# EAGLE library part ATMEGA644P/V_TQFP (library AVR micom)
ATMEGA644P TQFP pacage AVR micon series. producted by ATMEL.Co
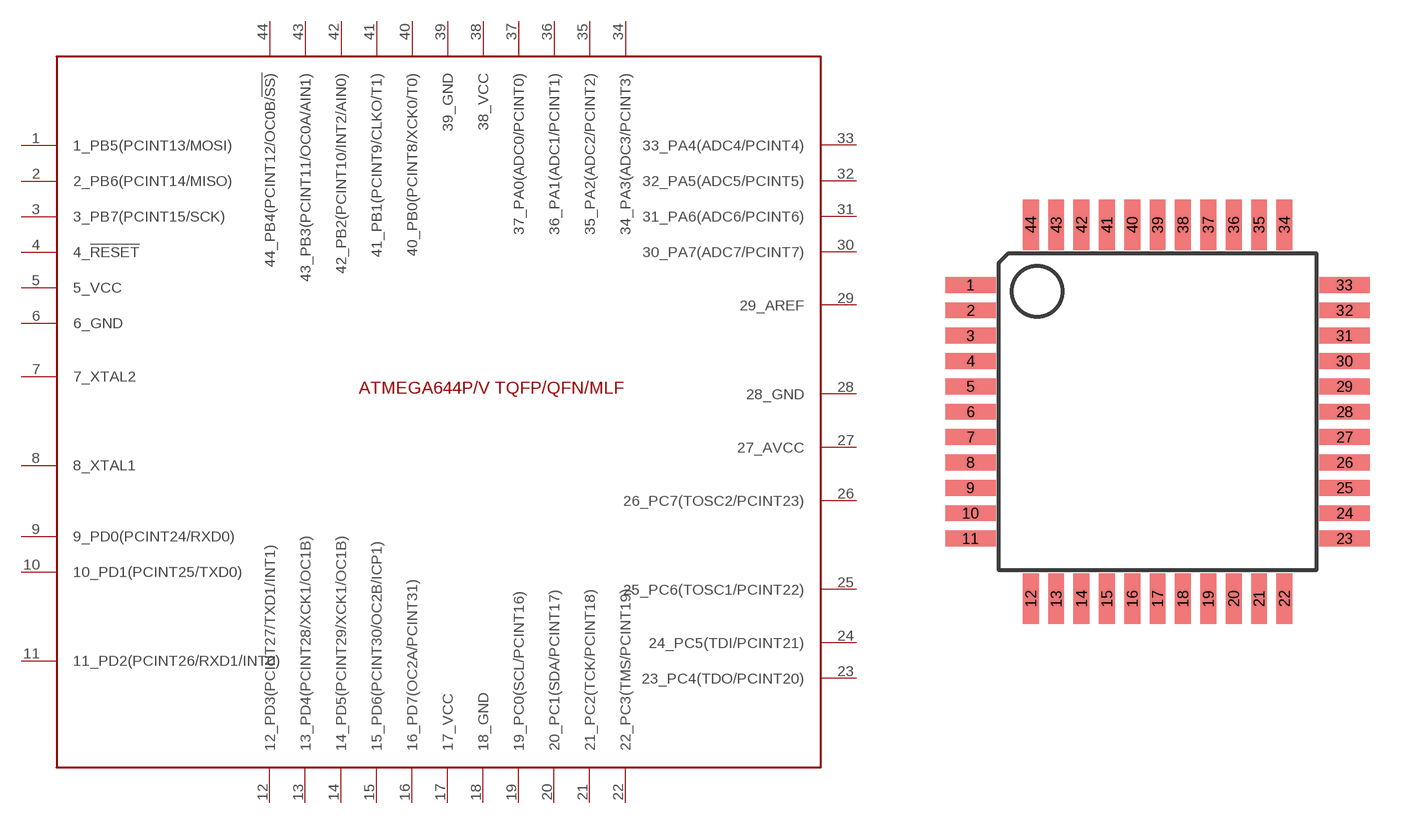
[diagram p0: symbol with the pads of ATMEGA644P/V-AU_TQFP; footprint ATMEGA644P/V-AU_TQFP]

Designator prefix U

## ATMEGA644P/V_TQFP  [ATMEGA644P/V-AU_TQFP]
1  1_PB5(PCINT13/MOSI)
2  2_PB6(PCINT14/MISO)
3  3_PB7(PCINT15/SCK)
4  4_!RESET
5  5_VCC
6  6_GND
7  7_XTAL2
8  8_XTAL1
9  9_PD0(PCINT24/RXD0)
10  10_PD1(PCINT25/TXD0)
11  11_PD2(PCINT26/RXD1/INT0)
12  12_PD3(PCINT27/TXD1/INT1)
13  13_PD4(PCINT28/XCK1/OC1B)
14  14_PD5(PCINT29/XCK1/OC1B)
15  15_PD6(PCINT30/OC2B/ICP1)
16  16_PD7(OC2A/PCINT31)
17  17_VCC
18  18_GND
19  19_PC0(SCL/PCINT16)
20  20_PC1(SDA/PCINT17)
21  21_PC2(TCK/PCINT18)
22  22_PC3(TMS/PCINT19)
23  23_PC4(TDO/PCINT20)
24  24_PC5(TDI/PCINT21)
25  25_PC6(TOSC1/PCINT22)
26  26_PC7(TOSC2/PCINT23)
27  27_AVCC
28  28_GND
29  29_AREF
30  30_PA7(ADC7/PCINT7)
31  31_PA6(ADC6/PCINT6)
32  32_PA5(ADC5/PCINT5)
33  33_PA4(ADC4/PCINT4)
34  34_PA3(ADC3/PCINT3)
35  35_PA2(ADC2/PCINT2)
36  36_PA1(ADC1/PCINT1)
37  37_PA0(ADC0/PCINT0)
38  38_VCC
39  39_GND
40  40_PB0(PCINT8/XCK0/T0)
41  41_PB1(PCINT9/CLKO/T1)
42  42_PB2(PCINT10/INT2/AIN0)
43  43_PB3(PCINT11/OC0A/AIN1)
44  44_PB4(PCINT12/OC0B/!SS)

## Footprint ATMEGA644P/V-AU_TQFP (pad centres in mm)
ATMEGA644P/V 10AU/20AU 44A(TQFN) pacage AVR micon series. producted by ATMEL.Co
smd 1.6 x 0.5: 1 -5.9,4; 2 -5.9,3.2; 3 -5.9,2.4; 4 -5.9,1.6; 5 -5.9,0.8; 6 -5.9,0; 7 -5.9,-0.8; 8 -5.9,-1.6; 9 -5.9,-2.4; 10 -5.9,-3.2; 11 -5.9,-4; 23 5.9,-4; 24 5.9,-3.2; 25 5.9,-2.4; 26 5.9,-1.6; 27 5.9,-0.8; 28 5.9,0; 29 5.9,0.8; 30 5.9,1.6; 31 5.9,2.4; 32 5.9,3.2; 33 5.9,4
smd 0.5 x 1.6: 12 -4,-5.9; 13 -3.2,-5.9; 14 -2.4,-5.9; 15 -1.6,-5.9; 16 -0.8,-5.9; 17 0,-5.9; 18 0.8,-5.9; 19 1.6,-5.9; 20 2.4,-5.9; 21 3.2,-5.9; 22 4,-5.9; 34 4,5.9; 35 3.2,5.9; 36 2.4,5.9; 37 1.6,5.9; 38 0.8,5.9; 39 0,5.9; 40 -0.8,5.9; 41 -1.6,5.9; 42 -2.4,5.9; 43 -3.2,5.9; 44 -4,5.9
